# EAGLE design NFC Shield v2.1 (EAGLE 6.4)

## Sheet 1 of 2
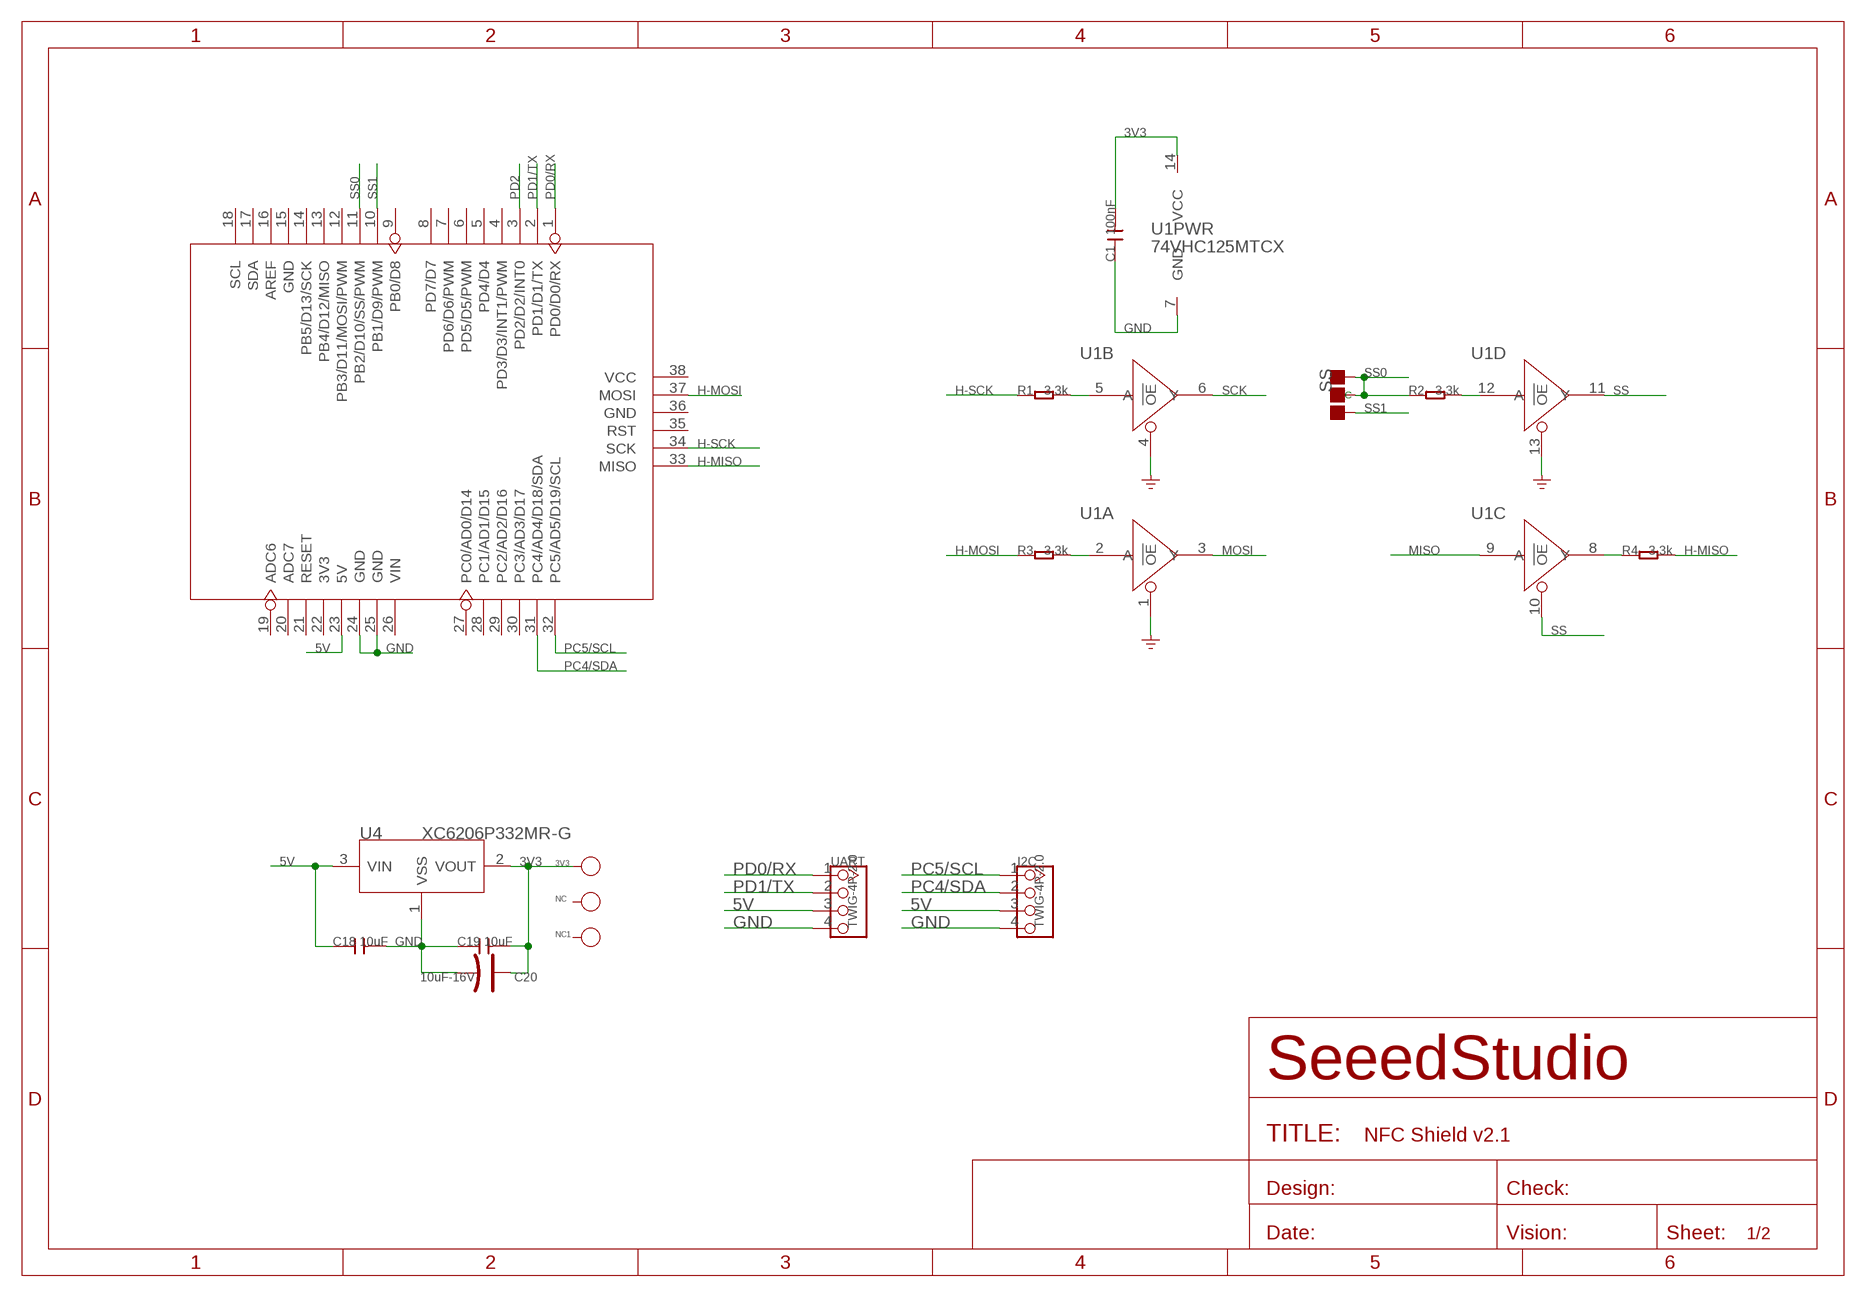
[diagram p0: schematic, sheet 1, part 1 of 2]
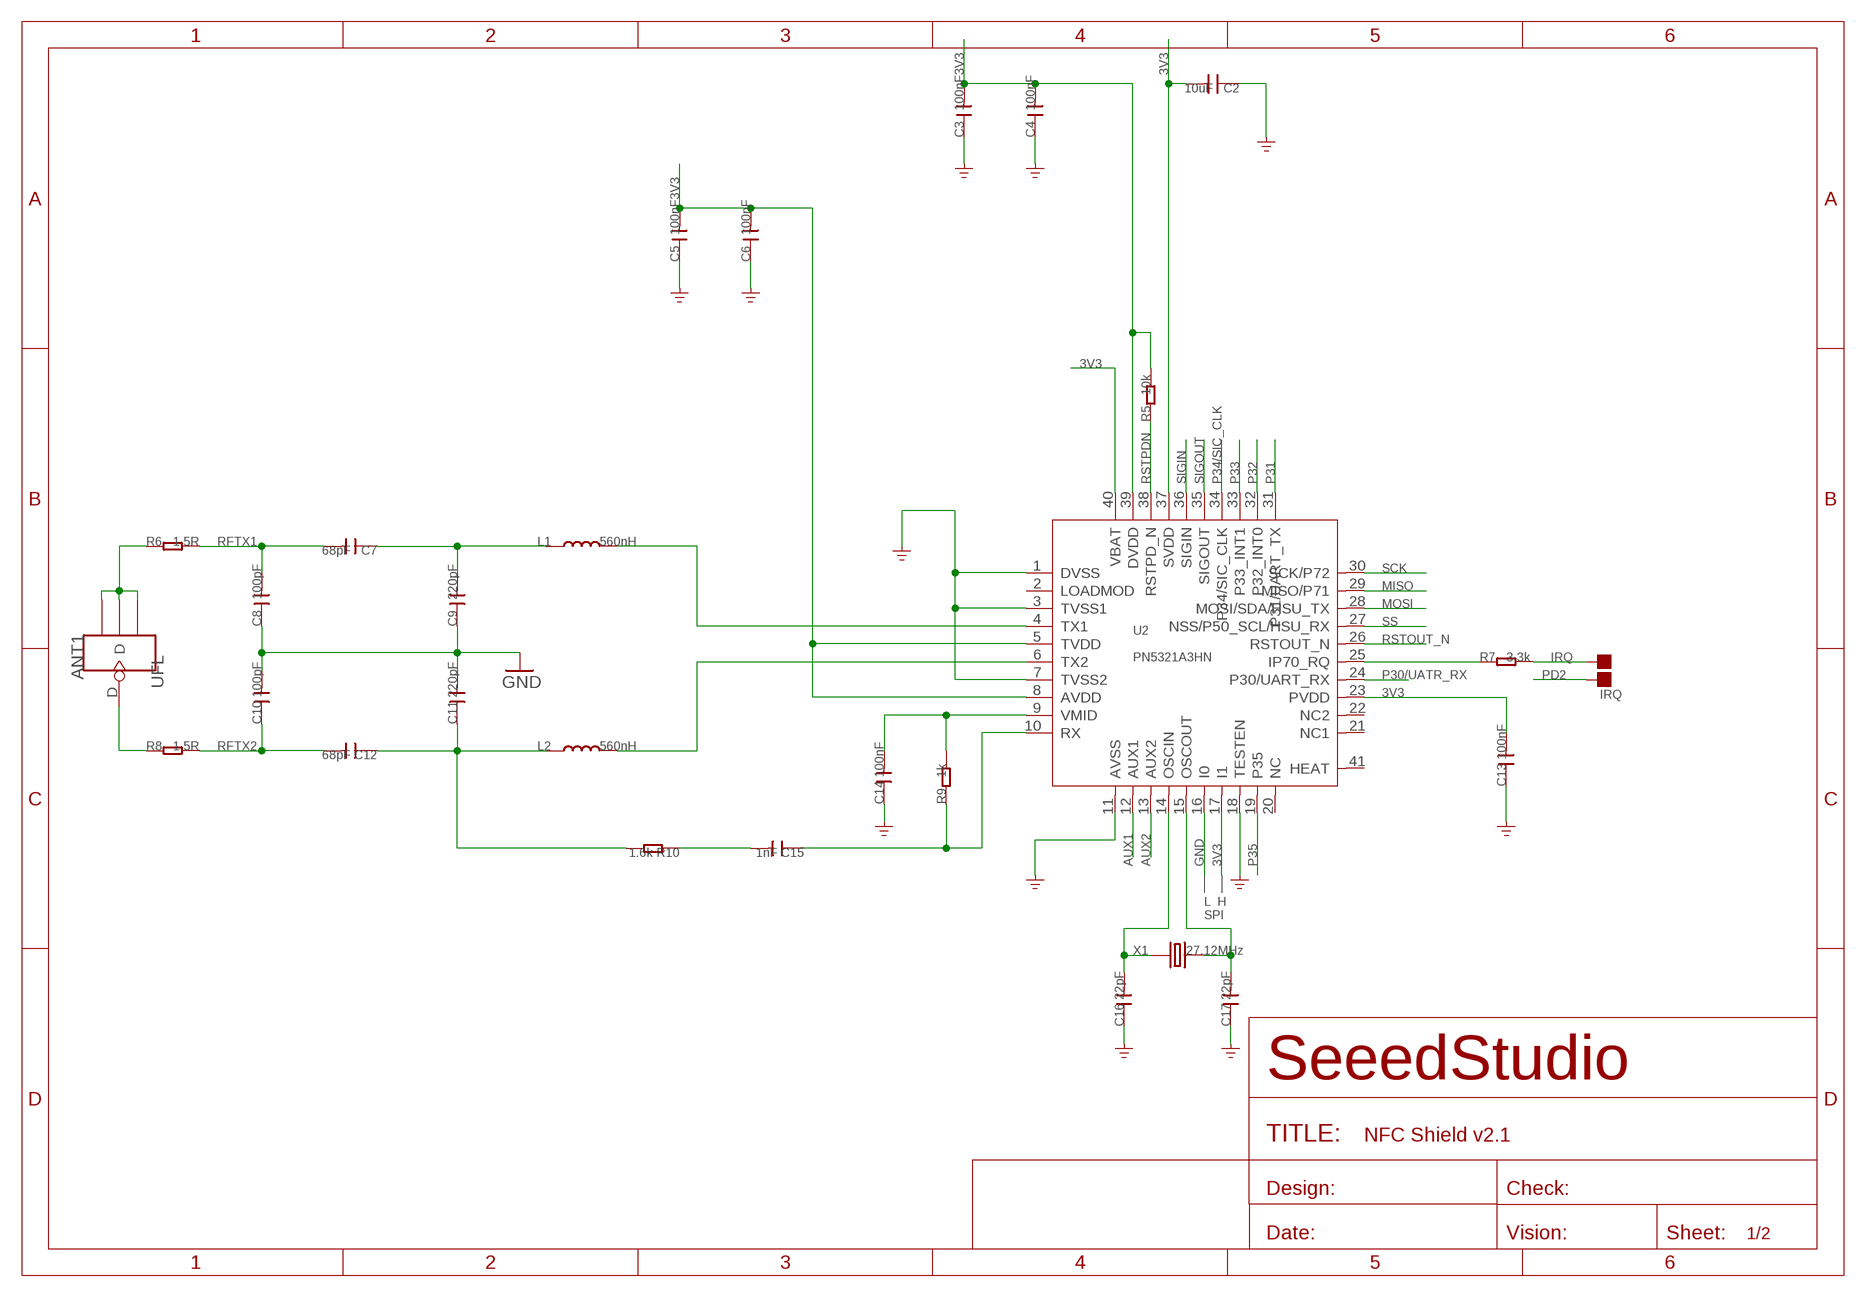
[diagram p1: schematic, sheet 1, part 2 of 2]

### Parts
3V3  DNP  PAD-TEST-POINT-CIRCLE'4545'  [TP_4545]
ANT1  UFL  ANTENNA-U-FL  [4P-U-FL]
C1  100nF  C-0603  [C0603]
C2  10uF  C-0805  [0805]
C3  100nF  C-0603  [C0603]
C4  100nF  C-0603  [C0603]
C5  100nF  C-0603  [C0603]
C6  100nF  C-0603  [C0603]
C7  68pF  C-0603  [C0603]
C8  100pF  C-0603  [C0603]
C9  220pF  C-0603  [C0603]
C10  100pF  C-0603  [C0603]
C11  220pF  C-0603  [C0603]
C12  68pF  C-0603  [C0603]
C13  100nF  C-0603  [C0603]
C14  100nF  C-0603  [C0603]
C15  1nF  C-0603  [C0603]
C16  22pF  C-0603  [C0603]
C17  22pF  C-0603  [C0603]
C18  10uF  C-0805  [C0805]
C19  10uF  C-0805  [C0805]
C20  10uF-16V  CAP-AVX-A  [AVX-A]
I2C  TWIG-4P-2.0  TWIG-4P-2.0-2.0  [4P-2.0]
IRQ  DNP  PAD-JUMPER-2P  [2P-SMD-1.78X1.27]
L1  560nH  L'0805'  [L0805]
L2  560nH  L'0805'  [L0805]
NC  DNP  PAD-TEST-POINT-CIRCLE'4545'  [TP_4545]
NC1  DNP  PAD-TEST-POINT-CIRCLE'4545'  [TP_4545]
R1  3.3k  R-0603  [R0603]
R2  3.3k  R-0603  [R0603]
R3  3.3k  R-0603  [R0603]
R4  3.3k  R-0603  [R0603]
R5  10k  R-0603  [R0603]
R6  1.5R  R-0603  [R0603]
R7  3.3k  R-0603  [R0603]
R8  1.5R  R-0603  [R0603]
R9  1k  R-0603  [R0603]
R10  1.6k  R-0603  [R0603]
SS  DNP  PAD-JUMPER-3P-40*40  [3P-SMD-4.1X1.5]
U1  74VHC125MTCX  74VHC125PW  [TSSOP14]
U2  PN5321A3HN  PN532-HVQFN40  [HVQFN40]
U4  XC6206P332MR-G  XC6206MR  [SOT23]
U5  ARDUINO-38P'WITH/-SILK'  [ARDUINO-38P-WITH/-SILK-500519002]
UART  TWIG-4P-2.0  TWIG-4P-2.0-2.0  [4P-2.0]
X1  27.12MHz  CRYSTAL'HC49S'  [HC49/S]

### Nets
3V3: 3V3.T C1.2 C2.2 C3.2 C4.2 C5.2 C6.2 C13.2 C19.2 C20.+ R5.2 U1.14(PWR:VCC) U2.5(TVDD) U2.8(AVDD) U2.17(I1) U2.23(PVDD) U2.37(SVDD) U2.39(DVDD) U2.40(VBAT) U4.2(VOUT)
5V: C18.1 I2C.3 U4.3(VIN) U5.23(5V) UART.3
AUX1: U2.12(AUX1)
AUX2: U2.13(AUX2)
GND: C1.1 C2.1 C3.1 C4.1 C5.1 C6.1 C8.1 C9.1 C10.2 C11.2 C13.1 C14.1 C16.1 C17.1 C18.2 C19.1 C20.- I2C.4 U1.1(A:!OE) U1.4(B:!OE) U1.7(PWR:GND) U1.13(D:!OE) U2.1(DVSS) U2.3(TVSS1) U2.7(TVSS2) U2.11(AVSS) U2.16(I0) U2.18(TESTEN) U4.1(VSS) U5.24(GND) U5.25(GND) UART.4
H-MISO: R4.2 U5.33(MISO)
H-MOSI: R3.1 U5.37(MOSI)
H-SCK: R1.1 U5.34(SCK)
IRQ: IRQ.1 R7.2
MISO: U1.9(C:A) U2.29(MISO/P71)
MOSI: U1.3(A:Y) U2.28(MOSI/SDA/HSU_TX)
N$1: C16.2 U2.14(OSCIN) X1.1
N$2: C17.2 U2.15(OSCOUT) X1.2
N$3: L2.2 U2.6(TX2)
N$4: L1.2 U2.4(TX1)
N$5: C7.1 C9.2 L1.1
N$6: C15.2 R10.1
N$7: C11.1 C12.1 L2.1 R10.2
N$8: R1.2 U1.5(B:A)
N$9: C14.2 R9.2 U2.9(VMID)
N$10: R2.2 U1.12(D:A)
N$11: C15.1 R9.1 U2.10(RX)
N$12: R4.1 U1.8(C:Y)
N$13: R3.2 U1.2(A:A)
N$14: R7.1 U2.25(IP70_RQ)
N$17: ANT1.D R8.1
N$18: ANT1.GND1 ANT1.GND2 ANT1.GND3 R6.1
P30/UATR_RX: U2.24(P30/UART_RX)
P31: U2.31(P31/UART_TX)
P32: U2.32(P32_INT0)
P33: U2.33(P33_INT1)
P34/SIC_CLK: U2.34(P34/SIC_CLK)
P35: U2.19(P35)
PC4/SDA: I2C.2 U5.31(PC4/AD4/D18/SDA)
PC5/SCL: I2C.1 U5.32(PC5/AD5/D19/SCL)
PD0/RX: U5.1(PD0/D0/RX) UART.1
PD1/TX: U5.2(PD1/D1/TX) UART.2
PD2: IRQ.2 U5.3(PD2/D2/INT0)
RFTX1: C7.2 C8.2 R6.2
RFTX2: C10.1 C12.2 R8.2
RSTOUT_N: U2.26(RSTOUT_N)
RSTPDN: R5.1 U2.38(RSTPD_N)
SCK: U1.6(B:Y) U2.30(SCK/P72)
SIGIN: U2.36(SIGIN)
SIGOUT: U2.35(SIGOUT)
SS: U1.10(C:!OE) U1.11(D:Y) U2.27(NSS/P50_SCL/HSU_RX)
SS0: R2.1 SS.11(R) SS.MM(C) U5.11(PB2/D10/SS/PWM)
SS1: SS.00(L) U5.10(PB1/D9/PWM)
Unconnected: NC1.T NC.T U2.2(LOADMOD) U2.20(NC) U2.21(NC1) U2.22(NC2) U2.41(HEAT) U5.4(PD3/D3/INT1/PWM) U5.5(PD4/D4) U5.6(PD5/D5/PWM) U5.7(PD6/D6/PWM) U5.8(PD7/D7) U5.9(PB0/D8) U5.12(PB3/D11/MOSI/PWM) U5.13(PB4/D12/MISO) U5.14(PB5/D13/SCK) U5.15(GND) U5.16(AREF) U5.17(SDA) U5.18(SCL) U5.19(ADC6) U5.20(ADC7) U5.21(RESET) U5.22(3V3) U5.26(VIN) U5.27(PC0/AD0/D14) U5.28(PC1/AD1/D15) U5.29(PC2/AD2/D16) U5.30(PC3/AD3/D17) U5.35(RST) U5.36(GND) U5.38(VCC)

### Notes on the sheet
- L | H
- SPI

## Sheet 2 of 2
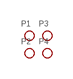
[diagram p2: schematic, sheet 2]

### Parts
P1  PAD-MARK  [ROUND-MARK-1.0]
P2  PAD-MARK  [ROUND-MARK-1.0]
P3  PAD-MARK  [ROUND-MARK-1.0]
P4  PAD-MARK  [ROUND-MARK-1.0]

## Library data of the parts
3V3 NC NC1 = Discrete:PAD-TEST-POINT-CIRCLE; PARTNO: DNP
ANT1 = Connector:ANTENNA-U-FL
C1 C3-C19 = Discrete:C*: Ceramic Capacitors
C2 = Discreter:C*: Ceramic Capacitors
C20 = Discrete:CAP*: Electrolytic Capacitors,Tantalum Capacitors and Super Capacitors
I2C UART = Connector:TWIG-4P-2.0
IRQ = Discrete:PAD-JUMPER-2P; PARTNO: DNP
L1 L2 = Discrete:L*
P1-P4 = Discrete:PAD-MARK; PARTNO: DNP
R1-R10 = Discrete:R*
SS = Discrete:PAD-JUMPER-3P; PARTNO: DNP
U1 = IC:74V*125: Quad Buffer/Line Driver;3-state
U2 = IC:PN532: NFC Controller http://www.adafruit.com/datasheets/pn532ds.pdf
U4 = IC:XC6206: LOW ESR Cap.Compatible Positive Voltage Regulators
U5 = moudle:ARDUINO-38P
X1 = Discrete:CRYSTAL*: CRYSTAL

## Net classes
0 default: width 0.203 mm, drill 0.305 mm, clearance 0.152 mm
3 usbvcc: width 0.203 mm, drill 0.305 mm, clearance 0.203 mm

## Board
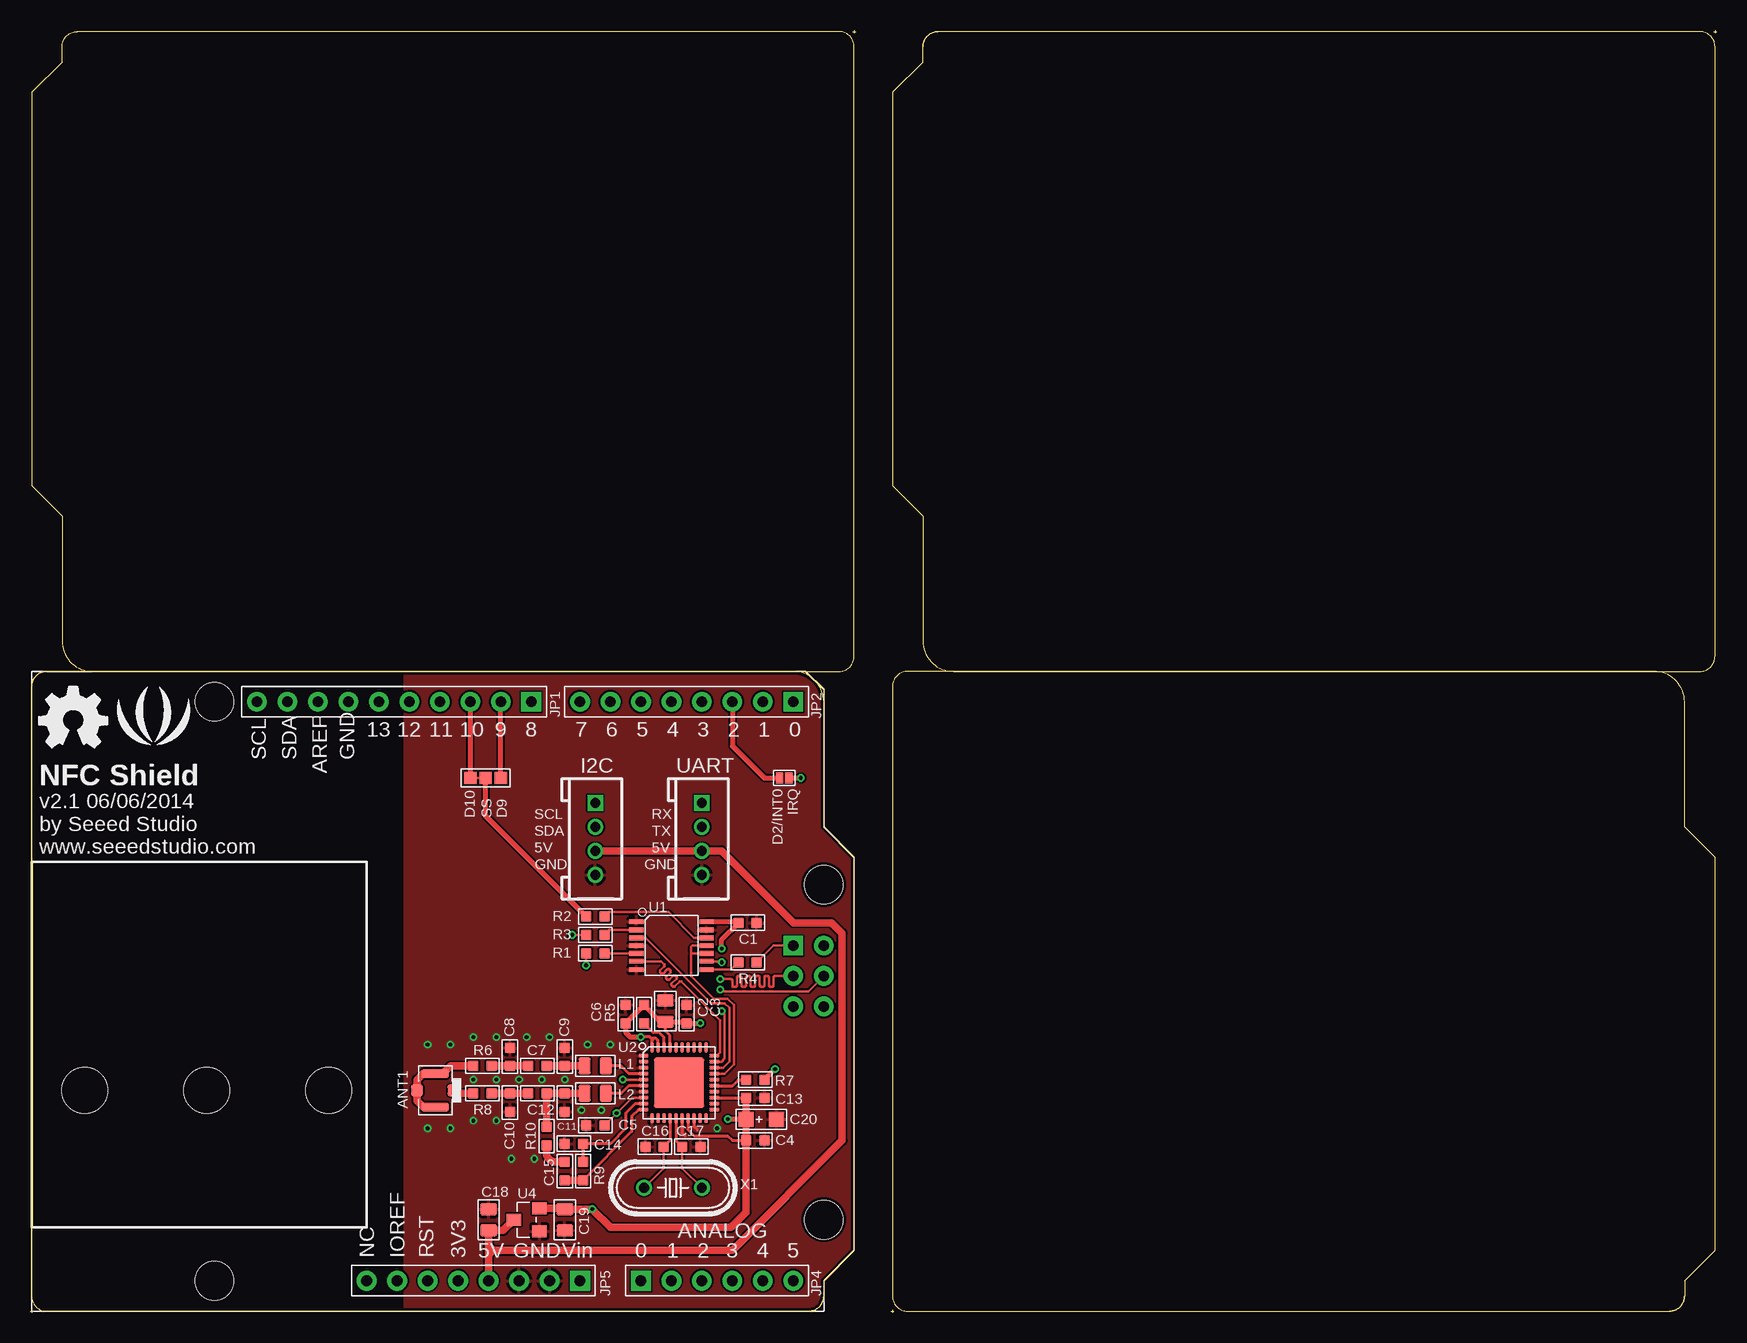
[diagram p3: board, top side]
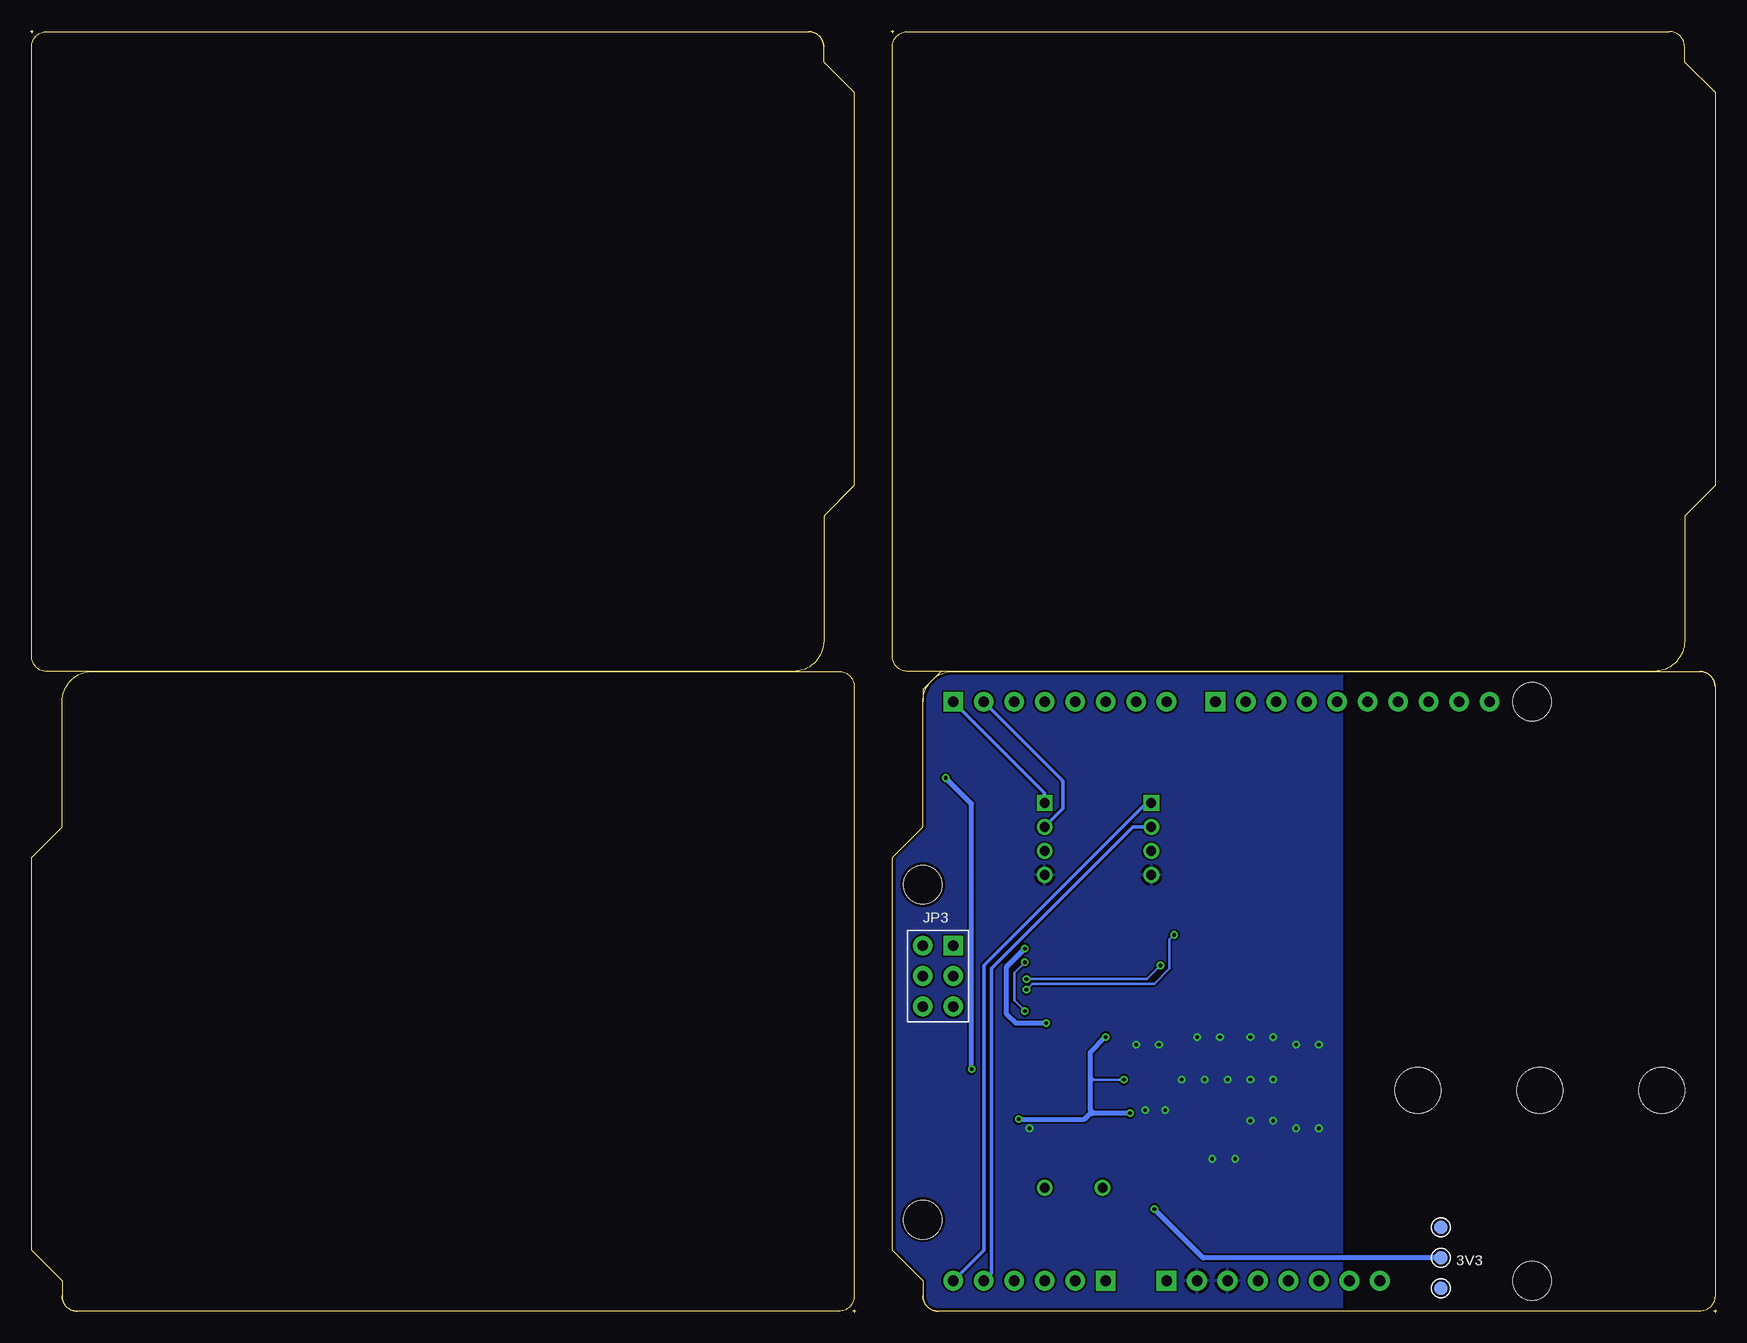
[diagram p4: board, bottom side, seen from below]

Size 140.59 x 106.93 mm. Coordinates in mm from the lower left corner, seen from the top.
Outline: 79 segments
Copper layers (1*16): Top 0.035mm / dielectric 1.5mm / Bottom 0.035mm
Design rules "SeeedStudio_rule_no_angle_090911 *": minimum track width 6mil, minimum drill 12mil, track to track 6mil, track to pad 6mil, pad to pad 6mil, via to via 6mil, smd to smd 0mil, copper to edge 10mil, drill to drill 10mil, minimum pad ring 10mil, minimum via ring 6mil, stop-mask expansion 2mil, vias tented up to drill 100mil, thermal gap 10mil
Holes 3.81 mm at 24.89,18.54 14.73,18.54 4.57,18.54
Holes 3.2 mm at 15.37,2.67
Holes 2.03 mm at 7.75,111.25 132.84,111.25 132.84,-4.32 7.75,-4.32
tRestrict: area 0.1,0.1 to 30.6,33.1; area 51.6,16.6 to 56.6,21.7
bRestrict: area 0.1,0.1 to 30.6,33.1

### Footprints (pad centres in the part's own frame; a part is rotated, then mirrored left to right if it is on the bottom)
TP_4545 = smd 1.143 x 1.143: T 0,0
4P-U-FL = smd 1.016 x 1.016: D -1.524,0; GND3 1.524,0 | smd 2.286 x 0.762: GND1 0,1.397; GND2 0,-1.397
C0603 = smd 0.889 x 0.889: 1 -0.762,0; 2 0.762,0
0805 = smd 1.016 x 1.397: 1 -0.889,0; 2 0.889,0
C0805 = smd 1.016 x 1.397: 1 -0.889,0; 2 0.889,0
AVX-A = smd 1.27 x 1.27: + -1.27,0; - 1.27,0
4P-2.0 = drill 0.8 pad 1.27 square: 1 -3,0 | drill 0.8 pad 1.27: 2 -1,0; 3 1,0; 4 3,0
2P-SMD-1.78X1.27 = smd 0.889 x 0.61: 1 0,0.381; 2 0,-0.381
L0805 = smd 1.016 x 1.397: 1 -0.889,0; 2 0.889,0
ROUND-MARK-1.0 = smd 1.016 x 1.016: P$1 0,0
R0603 = smd 0.889 x 0.889: 1 -0.762,0; 2 0.762,0
3P-SMD-4.1X1.5 = smd 1.016 x 1.016: 00 -1.27,0; 11 1.27,0; MM 0,0
TSSOP14 = smd 0.4 x 1.2: 1 -2,-2.925; 2 -1.3,-2.925; 3 -0.65,-2.925; 4 0,-2.925; 5 0.65,-2.925; 6 1.3,-2.925; 7 2,-2.925; 8 2,2.925; 9 1.3,2.925; 10 0.65,2.925; 11 0,2.925; 12 -0.65,2.925; 13 -1.3,2.925; 14 -2,2.925
HVQFN40 = smd 0.8 x 0.3: 1 -2.95,2.25; 2 -2.95,1.75; 3 -2.95,1.25; 4 -2.95,0.75; 5 -2.95,0.25; 6 -2.95,-0.25; 7 -2.95,-0.75; 8 -2.95,-1.25; 9 -2.95,-1.75; 10 -2.95,-2.25; 21 2.95,-2.25; 22 2.95,-1.75; 23 2.95,-1.25; 24 2.95,-0.75; 25 2.95,-0.25; 26 2.95,0.25; 27 2.95,0.75; 28 2.95,1.25; 29 2.95,1.75; 30 2.95,2.25 | smd 0.3 x 0.8: 11 -2.25,-2.95; 12 -1.75,-2.95; 13 -1.25,-2.95; 14 -0.75,-2.95; 15 -0.25,-2.95; 16 0.25,-2.95; 17 0.75,-2.95; 18 1.25,-2.95; 19 1.75,-2.95; 20 2.25,-2.95; 31 2.25,2.95; 32 1.75,2.95; 33 1.25,2.95; 34 0.75,2.95; 35 0.25,2.95; 36 -0.25,2.95; 37 -0.75,2.95; 38 -1.25,2.95; 39 -1.75,2.95; 40 -2.25,2.95 | smd 4.2 x 4.2: 41 0,0
SOT23 = smd 1.016 x 1.2: 1 -0.95,-1.06; 2 0.95,-1.06; 3 0,1.06
ARDUINO-38P-WITH/-SILK-500519002 = drill 0.889 pad 1.651 square: 1 63.5,50.8; 9 41.656,50.8; 26 45.72,2.54; 27 50.8,2.54; 33 63.5,30.48 | drill 0.889 pad 1.651: 2 60.96,50.8; 3 58.42,50.8; 4 55.88,50.8; 5 53.34,50.8; 6 50.8,50.8; 7 48.26,50.8; 8 45.72,50.8; 10 39.116,50.8; 11 36.576,50.8; 12 34.036,50.8; 13 31.496,50.8; 14 28.956,50.8; 15 26.416,50.8; 16 23.876,50.8; 17 21.336,50.8; 18 18.796,50.8; 19 27.94,2.54; 20 30.48,2.54; 21 33.02,2.54; 22 35.56,2.54; 23 38.1,2.54; 24 40.64,2.54; 25 43.18,2.54; 28 53.34,2.54; 29 55.88,2.54; 30 58.42,2.54; 31 60.96,2.54; 32 63.5,2.54; 34 63.5,27.94; 35 63.5,25.4; 36 66.04,25.4; 37 66.04,27.94; 38 66.04,30.48 | hole 3.2: 15.24,50.8; 66.04,35.56; 66.04,7.62
HC49/S = drill 0.813: 1 -2.413,0; 2 2.413,0

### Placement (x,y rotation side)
3V3  22.99,4.57 0 bottom
ANT1  33.78,18.54 180 top
C1  59.82,32.51 180 top
C2  52.96,25.15 270 top
C3  54.74,24.89 270 top
C4  60.45,14.35 180 top
C5  47.12,15.62 0 top
C6  49.66,24.89 270 top
C7  42.29,20.57 180 top
C8  40.01,21.34 270 top
C9  44.58,21.34 270 top
C10  40.01,17.53 270 top
C11  44.58,17.53 270 top
C12  42.29,18.29 180 top
C13  60.45,17.91 180 top
C14  45.34,14.1 0 top
C15  44.58,11.81 90 top
C16  52.07,13.84 0 top
C17  55.12,13.84 180 top
C18  38.23,7.75 90 top
C19  44.58,7.75 90 top
C20  60.96,16.13 0 top
I2C  47.12,39.5 270 top
IRQ  62.87,44.58 270 top
L1  47.12,20.57 0 top
L2  47.12,18.29 0 top
NC  22.99,7.11 0 bottom
NC1  22.99,2.03 0 bottom
P1  not placed on the board
P2  not placed on the board
P3  not placed on the board
P4  not placed on the board
R1  47.12,29.97 0 top
R2  47.12,33.02 0 top
R3  47.12,31.5 0 top
R4  59.82,29.21 0 top
R5  51.18,24.89 90 top
R6  37.72,20.57 0 top
R7  60.45,19.43 0 top
R8  37.72,18.29 0 top
R9  46.1,11.81 90 top
R10  43.05,14.73 90 top
SS  37.97,44.58 180 top
U1  53.47,30.61 270 top
U2  54.1,19.18 0 top
U4  41.4,7.75 90 top
U5  0.13,0.13 0 top
U$1  [OSHW_FILLX200_NOTEXT]  0.76,47.12 0 top
U$2  [LOGO_SILK]  10.29,49.02 0 top
UART  56.01,39.5 270 top
X1  53.59,10.41 0 top

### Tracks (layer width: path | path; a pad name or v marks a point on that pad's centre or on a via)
3V3  (via drill 0.3 pad 0.64)
  Top 0.203: U2.8 50.19,17.93 v48.9,16.64 C5.2 | U2.5 v49.41,19.43 v49.4,19.43
  Top 0.254: U2.17 54.85,15.25 55.37,14.73 58.17,14.73 58.55,14.35 C4.2 | U2.37 53.35,23.1 52.96,23.49 C2.2 | U2.23 59.67,17.93 C13.2 | U2.40 51.85,22.65 | 51.85,22.65 51.85,22.77 arc45 51.82,22.86 51.78,22.9 | U2.39 52.35,22.65 arc45 52.32,22.74 52.2,22.86 52.01,22.86 | 52.01,22.86 51.87,22.86 arc-45 51.78,22.9 | 51.85,22.65 arc-45 51.89,22.74 52.01,22.86 | 51.78,22.9 51.69,22.99 v50.93,22.99
  Top 0.406: C20.+ v58.17,16.13 | v50.93,22.99 50.04,22.99 49.66,23.37 C6.2 R5.2 52.58,24.26 C2.2 54.61,24.26 C3.2 v55.88,24.13 | v57.66,30.35 57.66,31.11 C1.2 58.96,32.61 U1.14
  Top 0.61: U4.2 44.52,8.7 C19.2 v46.86,8.64 48.39,7.11 58.42,7.11 59.69,8.38 C4.2 C20.+ C13.2
  Bottom 0.203: v49.4,19.43 51.94,19.43 | 51.94,19.43 52.2,19.68 | 52.2,19.18 51.94,19.43
  Bottom 0.406: v58.17,16.13 52.71,16.13 52.2,16.64 | 52.2,16.89 52.2,19.18 52.2,19.68 52.2,21.72 v50.93,22.99 | v48.9,16.64 51.94,16.64 | 52.2,16.64 51.94,16.64 | 51.94,16.64 52.2,16.89 | 52.2,16.89 52.2,16.64 | v55.88,24.13 58.42,24.13 59.18,24.89 59.18,28.83 v57.66,30.35 | 3V3.T 42.8,4.57 v46.86,8.64
5V
  Top 0.61: U5.23 38.23,4.83 | 38.23,4.83 38.23,5.21 | 38.23,5.21 38.23,5.59 | 38.23,5.59 C18.1 39.45,6.86 U4.3 | I2C.3 UART.3 57.64,38.5 63.63,32.51 66.8,32.51 67.69,31.62 67.69,14.35 58.55,5.21 38.61,5.21 | 38.61,5.21 38.23,5.21 | 38.61,5.21 38.23,5.59 | 38.23,4.83 38.61,5.21
GND  (via drill 0.3 pad 0.64)
  Top 0.254: U2.16 54.35,14.99 54.61,14.73 | U2.18 55.35,15.51 55.63,15.24
  other vias: 57.28,15.37 35.05,22.35 44.58,19.43 42.67,19.43 40.77,19.43 38.86,19.43 36.96,19.43 36.96,22.99 45.97,16.89 47.62,16.89 48.39,22.35 46.48,22.35 43.31,22.99 41.4,22.99 38.86,22.99 33.15,22.35 33.15,15.37 35.05,15.37 36.96,16 38.86,16 42.04,12.83 40.13,12.83
  pour Top: 31.24,53.47 31.24,0.13 66.17,0.13 66.17,2.67 68.71,5.21 68.71,37.97 66.17,40.51 66.17,51.94 64.64,53.47
  pour Bottom: 31.24,53.47 31.24,0.13 66.17,0.13 66.17,2.67 68.71,5.21 68.71,37.97 66.17,40.51 66.17,51.94 64.64,53.47
H-MISO
  Top 0.203: U5.33 61.98,30.61 R4.2
H-MOSI  (via drill 0.3 pad 0.64)
  Top 0.203: U5.37 64.9,26.8 57.66,26.8 v57.53,26.92 | v45.21,31.5 R3.1
  Bottom 0.203: v57.53,26.92 57.02,27.43 46.86,27.43 45.59,28.7 45.59,31.11 v45.21,31.5
H-SCK  (via drill 0.3 pad 0.64)
  Top 0.203: v46.36,28.96 R1.1 | v57.53,27.81 58.42,27.81 arc-90 58.55,27.69 58.55,27.18 58.8,27.18 arc90 58.93,27.3 58.93,27.94 arc-90 59.05,28.07 59.18,28.07 arc-90 59.31,27.94 59.31,27.3 arc90 59.44,27.18 59.56,27.18 arc90 59.69,27.3 59.69,27.94 arc-90 59.82,28.07 59.94,28.07 arc-90 60.07,27.94 60.07,27.3 arc90 60.2,27.18 60.33,27.18 arc90 60.45,27.3 60.45,27.94 arc-90 60.58,28.07 60.71,28.07 arc-90 60.83,27.94 60.83,27.3 arc90 60.96,27.18 61.09,27.18 arc90 61.21,27.3 61.21,27.94 arc-90 61.34,28.07 61.47,28.07 arc-90 61.6,27.94 61.6,27.3 arc90 61.72,27.18 61.85,27.18 arc90 61.98,27.3 61.98,27.94 arc-90 62.1,28.07 U5.34
  Bottom 0.203: v57.53,27.81 47.5,27.81 v46.36,28.96
IRQ  (via drill 0.3 pad 0.64)
  Top 0.406: R7.2 v62.1,20.32 | IRQ.1 v64.26,44.58
  Bottom 0.406: v62.1,20.32 62.1,42.42 v64.26,44.58
MISO  (via drill 0.3 pad 0.64)
  Top 0.203: U2.29 57.63,20.93 57.91,21.21 57.91,24.89 v57.66,25.15 | U1.9 57.56,29.31 v57.66,29.21
  Bottom 0.203: v57.66,25.15 58.55,26.04 58.55,28.32 v57.66,29.21
MOSI
  Top 0.203: U2.28 57.77,20.43 58.29,20.95 58.29,25.4 57.91,25.78 56.77,25.78 51.29,31.26 U1.3
N$1
  Top 0.203: C16.2 52.83,12.14 arc-45 52.78,12.01 X1.1
  Top 0.254: U2.14 53.35,14.36 C16.2
N$2
  Top 0.203: C17.2 54.36,12.14 arc45 54.41,12.01 X1.2
  Top 0.254: U2.15 53.85,14.35 C17.2
N$3
  Top 0.254: U2.6 49.91,18.93 49.28,18.29 L2.2
N$4
  Top 0.254: U2.4 49.92,19.93 49.28,20.57 L1.2
N$5
  Top 0.61: L1.1 C9.2 C7.1
N$6
  Top 0.61: R10.1 43.05,13.34 arc90 43.82,12.57 C15.2
N$7
  Top 0.61: L2.1 C11.1 C12.1 R10.2
N$8
  Top 0.203: R1.2 47.89,29.96 U1.5
N$9
  Top 0.254: U2.9 50.45,17.43 49.66,16.64 49.66,15.37 48.39,14.1 C14.2
  Top 0.305: R9.2 C14.2
N$10
  Top 0.203: R2.2 48.26,33.4 53.21,33.4 55.36,31.26 U1.12
N$11
  Top 0.254: U2.10 50.71,16.93 50.16,16.38 50.16,15.11 R9.1
  Top 0.61: C15.1 R9.1
N$12
  Top 0.203: U1.8 58.45,28.61 R4.1
N$13
  Top 0.203: R3.2 48.29,31.91 U1.2
N$14
  Top 0.254: U2.25 58.55,18.93 59.05,19.43 R7.1
N$17
  Top 0.61: R8.1 35.56,18.29 ANT1.D
N$18
  Top 0.61: R6.1 35.05,20.57 34.42,19.94 ANT1.GND2 32.77,19.94 32.26,19.43 ANT1.GND3 32.26,17.65 32.77,17.14 ANT1.GND1
PC4/SDA
  Bottom 0.305: I2C.2 48.66,40.5 60.45,28.7 60.45,3.3 U5.31
PC5/SCL
  Bottom 0.305: I2C.1 47.55,42.5 49.66,40.39 61.09,28.96 61.09,5.21 U5.32
PD0/RX
  Bottom 0.305: UART.1 56.01,43.25 arc-45 56.04,43.34 U5.1
PD1/TX
  Bottom 0.305: UART.2 arc45 56,40.52 54.48,42.04 54.48,44.27 arc-45 54.52,44.36 U5.2
PD2
  Top 0.406: U5.3 58.55,47.24 61.21,44.58 IRQ.2
RFTX1
  Top 0.61: C7.2 C8.2 R6.2
RFTX2
  Top 0.61: C12.2 C10.1 R8.2
RSTPDN
  Top 0.254: U2.38 52.85,22.97 52.45,23.37 51.94,23.37 R5.1
SCK
  Top 0.203: U2.30 57.24,21.43 57.53,21.72 57.53,24.38 54.32,27.6 arc90 54.14,27.6 53.75,27.2 arc-90 53.57,27.2 53.49,27.28 arc-90 53.49,27.46 53.89,27.85 arc90 53.89,28.03 53.81,28.1 arc90 53.63,28.1 53.3,27.78 arc-90 53.12,27.78 53.05,27.85 arc-90 53.05,28.03 53.38,28.36 arc90 53.38,28.54 53.3,28.61 arc90 53.12,28.61 52.8,28.28 arc-90 52.62,28.28 52.54,28.36 arc-90 52.54,28.54 52.87,28.87 arc90 52.87,29.05 52.61,29.31 U1.6
SS
  Top 0.203: U2.27 57.9,19.93 58.67,20.7 58.67,25.64 58.16,26.16 57.02,26.16 55.12,28.07 55.12,29.83 | 55.12,30.1 55.12,29.83 | U1.10 55.25,29.96 | 55.25,29.96 55.12,30.08 55.12,30.48 55.25,30.61 U1.11 | 55.12,29.83 55.25,29.96
SS0
  Top 0.203: SS.11 SS.MM
  Top 0.406: U5.11 SS.11 | R2.1 37.97,41.4 SS.MM
SS1
  Top 0.406: SS.00 U5.10

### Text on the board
tPlace: NFC Shield | D2/INT0 | D10 | D9 | SCL | RX | SDA | TX | v2.1 06/06/2014 / by Seeed Studio / www.seeedstudio.com | 5V | 5V | GND | GND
